FUNCTION_BLOCK DriveTyp
VAR_INPUT
END_VAR
VAR_OUTPUT
END_VAR

IF devTimer.Q THEN
	devTimer ( IN := FALSE, PT := devSpeed );
	engine :=  NOT engine;
	IF engine = FALSE THEN
		steps := steps + 1;
	END_IF
ELSE
	devTimer ( IN := TRUE, PT := devSpeed );
END_IF

END_FUNCTION_BLOCK
